FUNCTION "SVOLG_COILS" : VOID
TITLE =DECOILING MANAGEMENT
AUTHOR : DM
VERSION : 0.1

BEGIN
NETWORK
TITLE =COIL ROTATION IN JOG
//CLOCKWISE
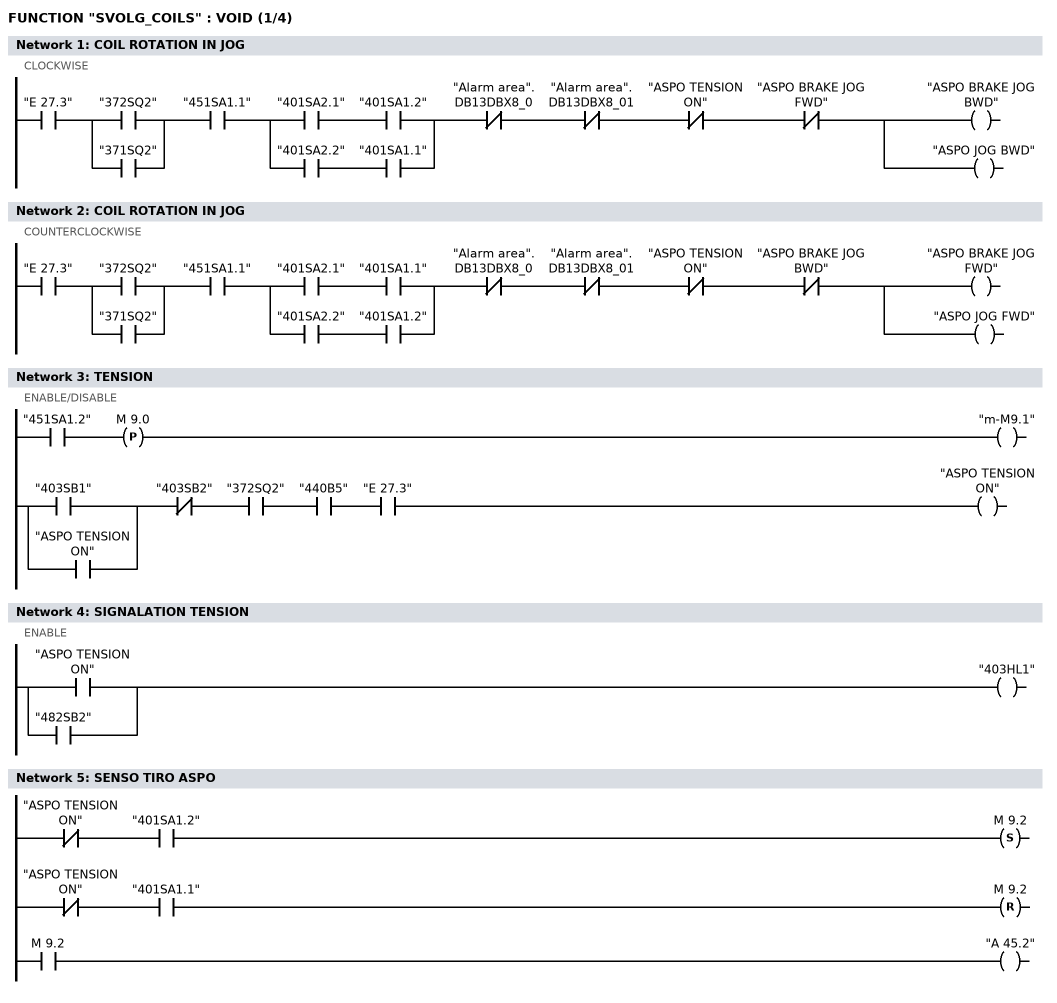
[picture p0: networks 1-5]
      U     "E      27.3";
      U(    ;
      O     "372SQ2";
      O     "371SQ2";
      )     ;
      U     "451SA1.1";
      U(    ;
      U     "401SA2.1";
      U     "401SA1.2";
      O     ;
      U     "401SA2.2";
      U     "401SA1.1";
      )     ;
      UN    "Alarm area".DB13DBX8_0;
      UN    "Alarm area".DB13DBX8_01;
      UN    "ASPO TENSION ON";
      UN    "ASPO BRAKE JOG FWD";

      =     "ASPO BRAKE JOG BWD";
      =     "ASPO JOG BWD";
NETWORK
TITLE =COIL ROTATION IN JOG
//COUNTERCLOCKWISE
      U     "E      27.3";
      U(    ;
      O     "372SQ2";
      O     "371SQ2";
      )     ;
      U     "451SA1.1";
      U(    ;
      U     "401SA2.1";
      U     "401SA1.1";
      O     ;
      U     "401SA2.2";
      U     "401SA1.2";
      )     ;
      UN    "Alarm area".DB13DBX8_0;
      UN    "Alarm area".DB13DBX8_01;
      UN    "ASPO TENSION ON";
      UN    "ASPO BRAKE JOG BWD";

      =     "ASPO BRAKE JOG FWD";
      =     "ASPO JOG FWD";
NETWORK
TITLE =TENSION
//ENABLE/DISABLE
      U     "451SA1.2";
      FP    M      9.0;
      =     "m-M9.1";

      U(    ;
      O     "403SB1";
      O     "ASPO TENSION ON";
      )     ;
      UN    "403SB2";
      U     "372SQ2";
      U     "440B5";
      U     "E      27.3";
      =     "ASPO TENSION ON";
NETWORK
TITLE =SIGNALATION TENSION
//ENABLE
      U     "ASPO TENSION ON";
      O     ;
      U     "482SB2";
      =     "403HL1";
NETWORK
TITLE =SENSO TIRO ASPO

      UN    "ASPO TENSION ON";
      U     "401SA1.2";
      S     M      9.2;
//;
      UN    "ASPO TENSION ON";
      U     "401SA1.1";
      R     M      9.2;
//;
      U     M      9.2;
      =     "A      45.2";

NETWORK
TITLE =RUN ASPO IN AUTOMATIC
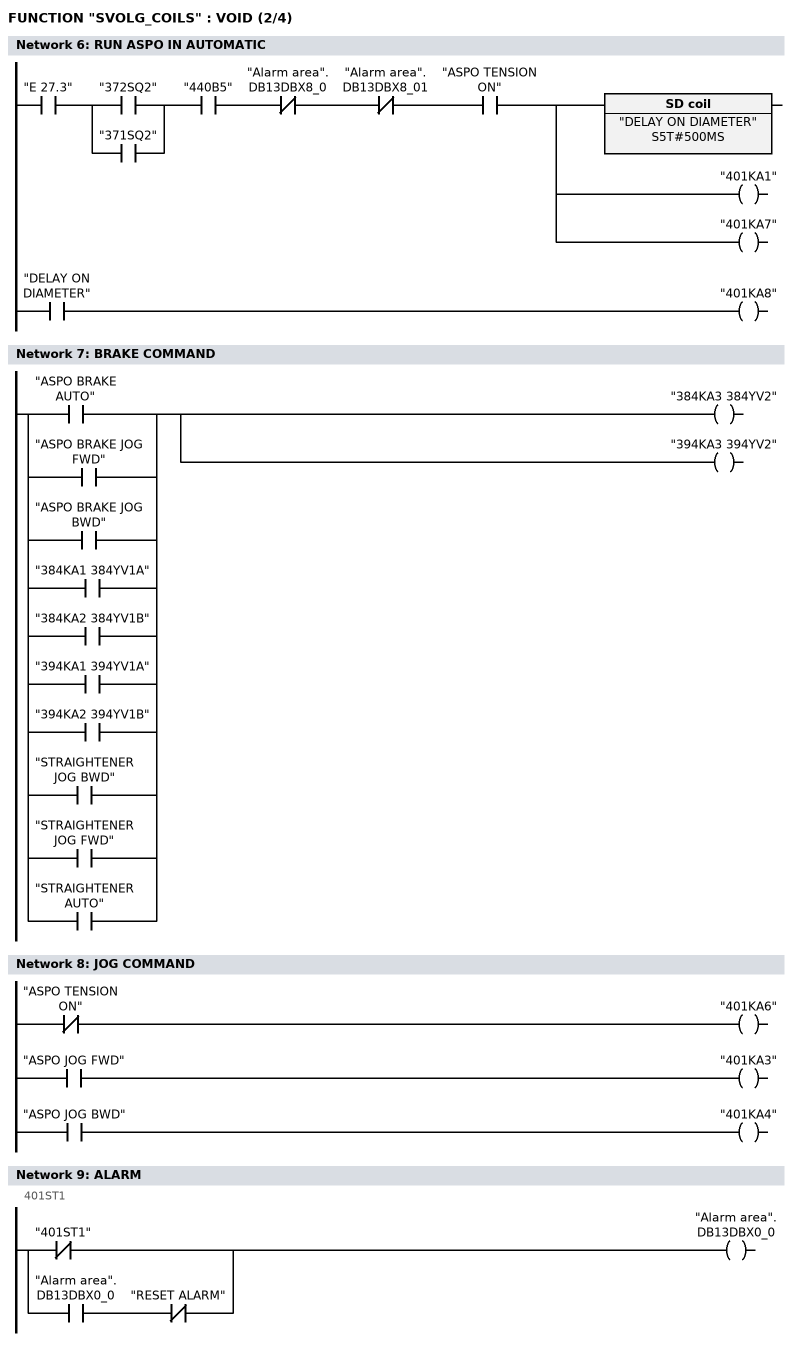
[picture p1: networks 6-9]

      U     "E      27.3";
      U(    ;
      O     "372SQ2";
      O     "371SQ2";
      )     ;
      U     "440B5";
      UN    "Alarm area".DB13DBX8_0;
      UN    "Alarm area".DB13DBX8_01;
      U     "ASPO TENSION ON";
      L     S5T#500MS;
      SE    "DELAY ON DIAMETER";
      =     "401KA1";
      =     "401KA7";

      U     "DELAY ON DIAMETER";
      =     "401KA8";
NETWORK
TITLE =BRAKE COMMAND

      O     "ASPO BRAKE AUTO";
      O     "ASPO BRAKE JOG FWD";
      O     "ASPO BRAKE JOG BWD";
      O     "384KA1 384YV1A";
      O     "384KA2 384YV1B";

      O     "394KA1 394YV1A";
      O     "394KA2 394YV1B";
      O     "STRAIGHTENER JOG BWD";
      O     "STRAIGHTENER JOG FWD";
      O     "STRAIGHTENER AUTO";
      =     "384KA3 384YV2";
      =     "394KA3 394YV2";
NETWORK
TITLE =JOG COMMAND

// JOG ENABLE
      UN    "ASPO TENSION ON";
      =     "401KA6";

// FORWARD
      U     "ASPO JOG FWD";
      =     "401KA3";

// BACKWARD
      U     "ASPO JOG BWD";
      =     "401KA4";

NETWORK
TITLE =ALARM
//401ST1
      UN    "401ST1";
      O     ;
      U     "Alarm area".DB13DBX0_0;
      UN    "RESET ALARM";
      =     "Alarm area".DB13DBX0_0;


NETWORK
TITLE =ALARM
//400KA2
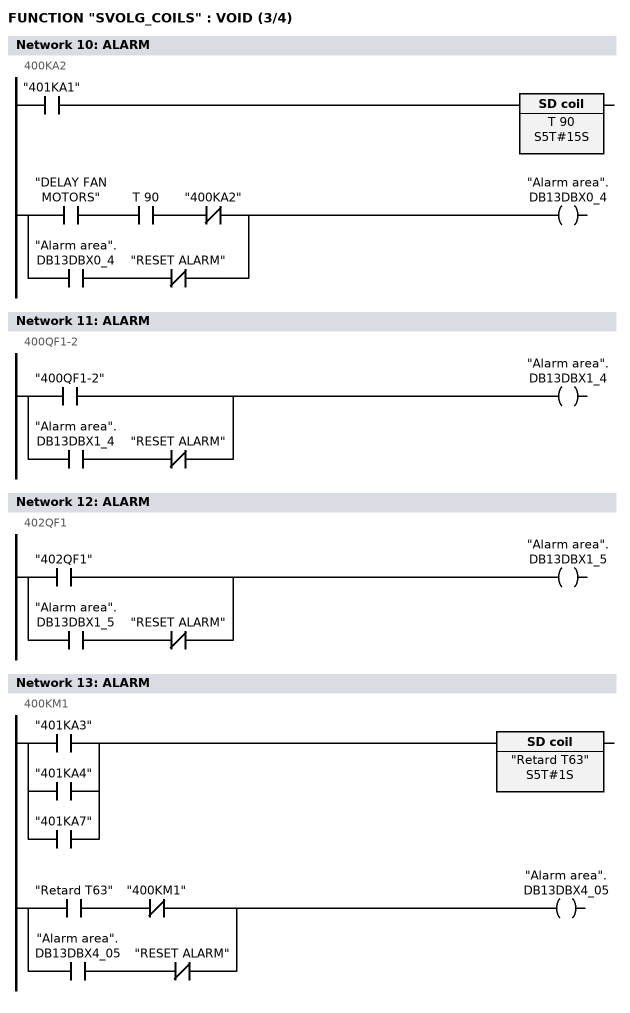
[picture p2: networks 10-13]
      U     "401KA1";
      L     S5T#15S;
      SE    T     90;

      U     "DELAY FAN MOTORS";
      U     T     90;
      UN    "400KA2";
      O     ;
      U     "Alarm area".DB13DBX0_4;
      UN    "RESET ALARM";
      =     "Alarm area".DB13DBX0_4;


NETWORK
TITLE =ALARM
//400QF1-2
      U     "400QF1-2";
      O     ;
      U     "Alarm area".DB13DBX1_4;
      UN    "RESET ALARM";
      =     "Alarm area".DB13DBX1_4;


NETWORK
TITLE =ALARM
//402QF1
      U     "402QF1";
      O     ;
      U     "Alarm area".DB13DBX1_5;
      UN    "RESET ALARM";
      =     "Alarm area".DB13DBX1_5;


NETWORK
TITLE =ALARM
//400KM1
      O     "401KA3";
      O     "401KA4";
      O     "401KA7";
      L     S5T#1S;
      SE    "Retard T63";

      U     "Retard T63";
      UN    "400KM1";
      O     ;
      U     "Alarm area".DB13DBX4_05;
      UN    "RESET ALARM";
      =     "Alarm area".DB13DBX4_05;

NETWORK
TITLE =ALARM
//400KM1
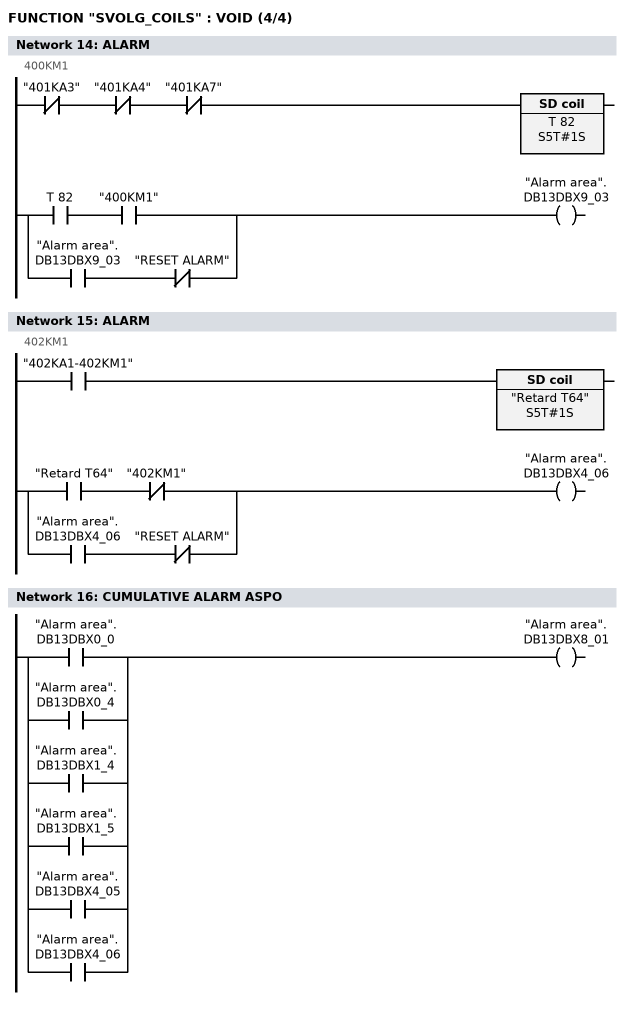
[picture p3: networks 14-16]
      UN    "401KA3";
      UN    "401KA4";
      UN    "401KA7";
      L     S5T#1S;
      SE    T     82;

      U     T     82;
      U     "400KM1";
      O     ;
      U     "Alarm area".DB13DBX9_03;
      UN    "RESET ALARM";
      =     "Alarm area".DB13DBX9_03;

NETWORK
TITLE =ALARM
//402KM1
      U     "402KA1-402KM1";
      L     S5T#1S;
      SE    "Retard T64";

      U     "Retard T64";
      UN    "402KM1";
      O     ;
      U     "Alarm area".DB13DBX4_06;
      UN    "RESET ALARM";
      =     "Alarm area".DB13DBX4_06;

NETWORK
TITLE =CUMULATIVE ALARM ASPO

      O     "Alarm area".DB13DBX0_0;
      O     "Alarm area".DB13DBX0_4;
      O     "Alarm area".DB13DBX1_4;
      O     "Alarm area".DB13DBX1_5;
      O     "Alarm area".DB13DBX4_05;
      O     "Alarm area".DB13DBX4_06;
      =     "Alarm area".DB13DBX8_01;

END_FUNCTION

